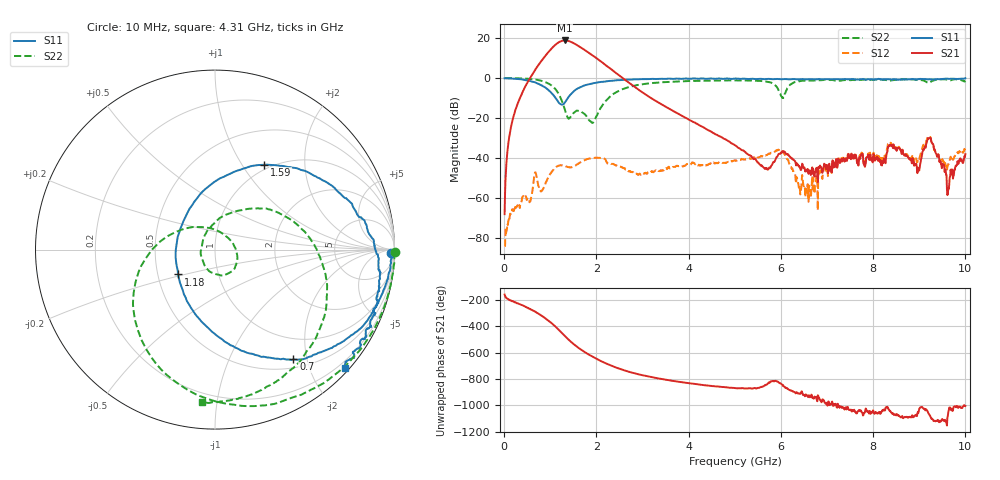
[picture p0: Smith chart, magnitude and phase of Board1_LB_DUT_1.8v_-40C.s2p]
! Created Tue May 27 15:57:59 2025
# hz S ma R 50
! 2 Port Network Data from SP1.SP block
! freq  magS11  angS11  magS21  angS21  magS12  angS12  magS22  angS22
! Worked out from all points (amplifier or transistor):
!   1000 points, 10 MHz to 10 GHz, reference 50 ohm
!   highest |S21| = 18.8 dB at 1.31 GHz (marker M1)
!   |S21| within 3 dB of that: 1.071 GHz to 1.63 GHz (558.3 MHz wide, 41.3 % of centre)
!   unconditionally stable (mu >= 1): 19.49 MHz to 24.01 MHz; 86.09 MHz to 109.9 MHz; 110.1 MHz to end of sweep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
!   at 1.67 GHz: K = 6.79, MAG = 17.3 dB, |S12| = -41.9 dB
!   at 5.01 GHz: K = 28.94, MAG = -13.8 dB, |S12| = -41.2 dB
!   at 10 GHz: K = 10.87, MAG = -15.1 dB, |S12| = -34.6 dB
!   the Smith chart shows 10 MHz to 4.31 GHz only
!   S11 on the Smith chart (normalised r, x): 10 MHz: 58, -59; 700 MHz: 0.63, -1.77; 1.18 GHz: 0.64, -0.19; 1.59 GHz: 0.94, +1.26; 4.31 GHz: 0.09, -2.58
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1e7  0.9833 -1.0  0.0003979 -162.3  6.305e-05 156.1  1.004 -0.8
1.9e8  0.9681 -12.9  0.09671 148.0  0.000527 78.8  0.9953 -17.1
7e8  0.7518 -54.4  1.789 62.3  0.003564 67.0  0.9122 -72.0
9.4e8  0.5269 -82.3  4.208 6.6  0.003027 113.2  0.751 -110.4
1.07e9  0.3742 -107.4  6.145 -30.9  0.005114 98.4  0.5937 -138.7
1.18e9  0.2484 -146.1  7.783 -67.2  0.006468 78.5  0.4048 -170.0
1.25e9  0.2164 174.1  8.477 -91.9  0.006576 67.9  0.2737 164.1
1.31e9  0.2384 136.8  8.709 -113.2  0.006377 60.6  0.173 133.0
1.44e9  0.3873 88.2  8.115 -156.6  0.00589 57.9  0.107 16.1
1.59e9  0.5465 59.9  6.581 160.7  0.007003 59.4  0.1531 -52.6
1.68e9  0.6138 48.6  5.648 138.5  0.008164 54.2  0.1426 -80.4
1.9e9  0.7312 30.3  3.801 91.6  0.01005 32.0  0.07735 -179.8
2.12e9  0.8042 17.9  2.495 51.6  0.01003 7.2  0.2009 73.6
2.54e9  0.8957 -0.3  1.066 -7.6  0.005998 -11.6  0.5119 10.9
3.34e9  0.9523 -21.6  0.2457 -75.5  0.004765 10.6  0.7725 -50.2
4.31e9  0.977 -42.3  0.05971 -125.8  0.006363 -3.1  0.854 -95.0
5.01e9  0.9763 -56.0  0.0209 -148.2  0.008744 -8.2  0.876 -119.4
6.67e9  0.94 -87.8  0.005255 159.1  0.002565 164.5  0.867 -150.6
8.34e9  0.9311 -132.9  0.01962 50.4  0.02241 55.3  0.8625 167.6
9.23e9  0.9333 -157.0  0.03139 5.9  0.03352 12.9  0.779 161.7
9.62e9  0.9612 -167.5  0.0013 3.7  0.006577 49.6  0.9014 152.8
1e10  0.9917 -179.4  0.0126 76.4  0.01863 68.8  0.8457 144.7
